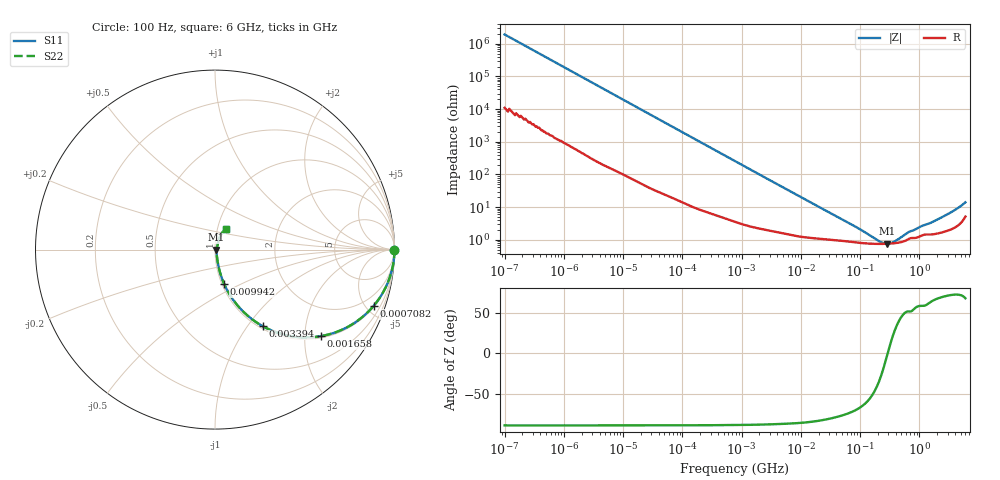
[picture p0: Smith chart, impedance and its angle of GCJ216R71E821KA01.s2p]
!Murata Part Number: GCJ216R71E821KA01
!These Parameters are Measured in Series Mode Connection
!Data Generated on Mar 13, 2026
!  o--ll--o
!Port1  Port2
!  o------o
!Operation Temp=25[degC], DC Bias Voltage=0[V]
!Freq. Start=100[Hz] Stop=6[GHz] 401[Steps]
# Hz S RI R 50
!Freq.(Hz) S11(Real) S11(Imag) S21(Real) S21(Imag) S12(Real) S12(Imag) S22(Real) S22(Imag)
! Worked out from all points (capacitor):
!   401 points, 100 Hz to 6 GHz, reference 50 ohm
!   read as one part in series: C = 827 pF near 109 Hz
!   lowest |Z| = 759 mohm at 285.7 MHz (marker M1)
!   series resonance near 292.7 MHz, so ESL is about 360 pH
!   S11 on the Smith chart (normalised r, x): 100 Hz: open; 708.2 kHz: 1.08, -5.61; 1.658 MHz: 1.05, -2.41; 3.394 MHz: 1.04, -1.18; 9.942 MHz: 1.02, -0.41; 6 GHz: 1.10, +0.26
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100  1 -5.2e-05  3e-07 5.2e-05  3e-07 5.2e-05  1 -5.2e-05
205  1 -0.000106  6e-07 0.000106  6e-07 0.000106  1 -0.000106
2008  1 -0.00103  5.9e-06 0.00103  5.9e-06 0.00103  1 -0.00103
40335  0.9995 -0.0206  0.000545 0.0206  0.000545 0.0206  0.9995 -0.0206
211427  0.9878 -0.1058  0.0122 0.1058  0.0122 0.1058  0.9878 -0.1058
432798  0.9523 -0.2076  0.0477 0.2076  0.0477 0.2076  0.9523 -0.2076
708247  0.8839 -0.3137  0.1161 0.3137  0.1161 0.3137  0.8839 -0.3137
774597  0.8647 -0.3352  0.1353 0.3352  0.1353 0.3352  0.8647 -0.3352
1658239  0.5901 -0.482  0.4099 0.482  0.4099 0.482  0.5901 -0.482
2372521  0.418 -0.4811  0.582 0.4811  0.582 0.4811  0.418 -0.4811
3394479  0.2659 -0.4267  0.7341 0.4267  0.7341 0.4267  0.2659 -0.4267
5554849  0.127 -0.3129  0.873 0.3129  0.873 0.3129  0.127 -0.3129
9941735  0.051 -0.1917  0.949 0.1917  0.949 0.1917  0.051 -0.1917
1.555665e7  0.0276 -0.1262  0.9724 0.1262  0.9724 0.1262  0.0276 -0.1262
8.154455e7  0.00892 -0.0242  0.9911 0.0242  0.9911 0.0242  0.00892 -0.0242
2.088084e8  0.00747 -0.00519  0.9925 0.00519  0.9925 0.00519  0.00747 -0.00519
2.856706e8  0.00752 -0.000366  0.9925 0.000366  0.9925 0.000366  0.00752 -0.000366
3.124326e8  0.00759 0.000993  0.9924 -0.000993  0.9924 -0.000993  0.00759 0.000993
3.908258e8  0.00788 0.00446  0.9921 -0.00446  0.9921 -0.00446  0.00788 0.00446
6.688484e8  0.0108 0.0135  0.9892 -0.0135  0.9892 -0.0135  0.0108 0.0135
2.679998e9  0.02 0.0497  0.98 -0.0497  0.98 -0.0497  0.02 0.0497
6e9  0.0635 0.1166  0.9365 -0.1166  0.9365 -0.1166  0.0635 0.1166
